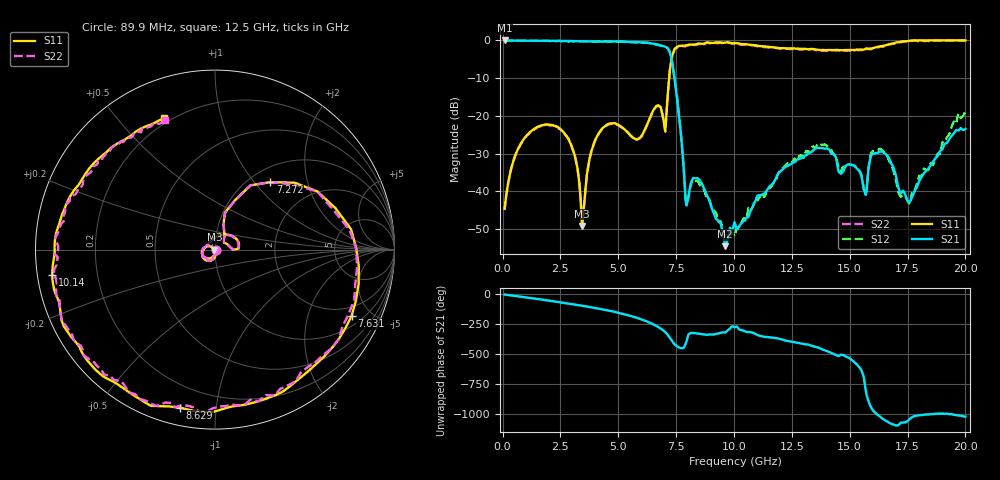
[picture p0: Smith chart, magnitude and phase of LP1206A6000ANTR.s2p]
!	AVX	THIN	FILM	OPERATION
!	LP1206	High	Performance	Low	Pass	Filters
!	P/N	LP1206A6000ANTR	11	February	2016
!	File	saved	on	"Wednesday,"	April	"05,"	2017	using	DaVinci	by	Abstraction	Software	Inc.	(c)	1998
#	MHZ	S	DB	R	50
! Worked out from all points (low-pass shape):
!   500 points, 89.9 MHz to 20 GHz, reference 50 ohm
!   highest |S21| = -0.01 dB at 89.9 MHz (marker M1); lowest = -54.6 dB at 9.626 GHz (marker M2)
!   |S21| within 3 dB of the highest: start of sweep to 7.221 GHz
!   lowest |S11| = -49.2 dB at 3.442 GHz (marker M3), VSWR 1.01, Z = 49.7 + j0.0129 ohm
!   |S11| at or under -10 dB: start of sweep to 7.201 GHz
!   |S22| runs from -49.2 to 0.0 dB; largest |S21 - S12| = 0.054
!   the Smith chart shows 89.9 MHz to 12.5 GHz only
!   S11 on the Smith chart (normalised r, x): 89.9 MHz: 1.01, -0.01; 7.272 GHz: 1.23, +1.21; 7.631 GHz: 1.46, -3.81; 8.629 GHz: 0.08, -0.80; 10.14 GHz: 0.04, -0.08; 12.5 GHz: 0.18, +0.67
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89.9  -44.70 -31.8  -0.01 -2.5  0.00 -2.1  -44.90 -31.8
728.3  -28.07 -104.2  -0.07 -19.1  -0.07 -19.2  -28.27 -104.3
1965.2  -22.31 -160.3  -0.09 -52.2  -0.09 -52.4  -22.31 -160.5
2922.8  -27.11 153.9  -0.17 -80.1  -0.17 -80.0  -27.11 153.7
3441.5  -49.20 177.8  -0.21 -96.3  -0.20 -96.0  -49.20 177.8
4159.7  -24.62 -104.0  -0.29 -120.6  -0.23 -121.2  -24.72 -104.2
5516.3  -25.11 167.2  -0.38 179.2  -0.47 179.0  -25.21 167.2
6753.2  -17.26 11.3  -1.24 82.6  -1.10 81.9  -17.46 11.2
7032.5  -24.09 41.1  -1.66 42.7  -1.63 40.8  -24.19 40.9
7271.9  -6.26 50.6  -4.15 -15.4  -4.13 -14.8  -6.26 50.5
7631  -1.45 -26.0  -20.25 -86.4  -20.15 -84.8  -1.65 -26.1
7950.2  -1.30 -58.3  -43.79 -34.5  -43.42 -33.7  -1.30 -58.4
8628.5  -0.90 -102.6  -38.21 25.1  -39.07 28.9  -1.00 -102.6
9626  -0.56 -149.1  -54.59 39.6  -51.68 47.9  -0.66 -149.1
10064.9  -0.70 -167.4  -49.04 86.4  -51.08 71.8  -0.90 -167.5
10144.7  -0.74 -171.1  -50.11 86.6  -49.60 63.9  -0.84 -171.3
12498.8  -2.10 111.3  -32.61 -37.2  -32.39 -33.3  -2.20 111.1
13376.6  -2.27 83.6  -29.42 -72.2  -28.29 -68.0  -2.27 83.5
15650.9  -2.30 19.0  -40.22 -28.9  -40.20 -33.1  -2.40 18.9
16688.3  -1.06 -12.5  -31.18 5.8  -31.71 8.8  -1.06 -12.5
17566.1  -0.11 -46.3  -42.77 29.8  -43.18 34.1  -0.11 -46.5
20000  0.00 -128.8  -23.49 55.2  -18.75 40.1  0.00 -128.8
